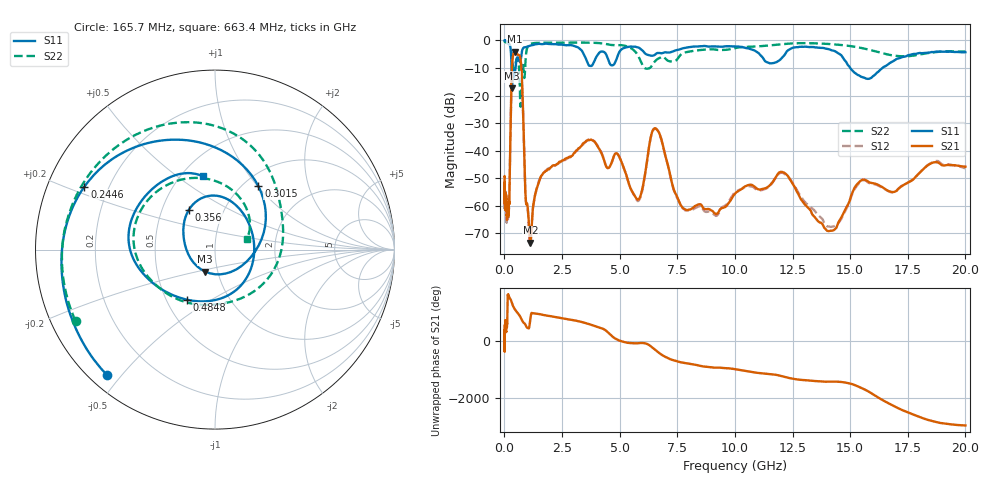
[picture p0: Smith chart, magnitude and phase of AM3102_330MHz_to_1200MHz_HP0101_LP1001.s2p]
! Date/Time: Tue, Sep 11, 2018 5:14 PM
! Network Analyzer: Agilent Technologies E8362B Rev: A.07.50.63
! Sweep from 0.010 to 20.000 GHz, 1601 Points, Sweep Type: LOG
! Power Supply: 4.949 V, 0.001 A
# Hz S DB R 50
!freq MagS11 AngS11 MagS21 AngS21 MagS12 AngS12 MagS22 AngS22
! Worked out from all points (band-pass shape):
!   1601 points, 10 MHz to 20 GHz, reference 50 ohm
!   highest |S21| = -4.09 dB at 455.8 MHz (marker M1); lowest = -73.4 dB at 1.129 GHz (marker M2)
!   |S21| within 3 dB of the highest: 347.4 MHz to 706.1 MHz (358.8 MHz wide, 68.1 % of centre)
!   lowest |S11| = -17.4 dB at 331.5 MHz (marker M3), VSWR 1.31, Z = 43.6 - j10.9 ohm
!   |S11| at or under -10 dB: 309.7 MHz to 483.4 MHz (173.8 MHz wide, 43.8 % of centre); 15.01 GHz to 16.41 GHz (1.4 GHz wide, 8.91 % of centre)
!   |S22| runs from -24.1 to -0.3 dB; largest |S21 - S12| = 0.012
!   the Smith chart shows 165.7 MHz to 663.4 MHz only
!   S11 on the Smith chart (normalised r, x): 165.7 MHz: 0.05, -0.46; 244.6 MHz: 0.11, +0.23; 301.5 MHz: 1.17, +1.01; 356 MHz: 0.68, +0.32; 484.8 MHz: 0.63, -0.39; 663.4 MHz: 0.63, +0.62
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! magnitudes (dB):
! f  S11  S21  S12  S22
! 10 MHz  0.0  -49.2  -53.5  -0.3
! 35.55 MHz  0.0  -60.4  -59.1  -0.5
! 126.4 MHz  -0.4  -64.1  -63.2  -1.0
! 165.7 MHz  -0.7  -62.3  -64.4  -1.2
! 244.6 MHz  -1.9  -43.2  -43.3  -1.8
! 301.5 MHz  -7.4  -17.4  -17.4  -3.6
! 331.5 MHz  -17.4  -9.0  -9.0  -6.4
! 356 MHz  -11.5  -6.5  -6.6  -8.3
! 447.2 MHz  -12.1  -4.1  -4.1  -9.5
! 455.8 MHz  -11.6  -4.1  -4.1  -9.2
! 484.8 MHz  -9.9  -4.2  -4.2  -8.3
! 663.4 MHz  -7.6  -5.6  -5.6  -14.5
! 925.1 MHz  -2.5  -57.4  -57.5  -6.3
! 1.129 GHz  -1.9  -73.4  -74.4  -1.3
! 1.59 GHz  -1.3  -49.3  -49.4  -0.8
! 3.757 GHz  -9.3  -36.0  -35.9  -0.8
! 5.652 GHz  -2.3  -56.4  -56.7  -3.9
! 6.549 GHz  -5.1  -31.9  -32.1  -7.4
! 7.845 GHz  -2.7  -61.4  -61.7  -4.4
! 12.09 GHz  -5.9  -47.9  -48.1  -1.3
! 14.01 GHz  -3.1  -69.1  -67.5  -1.3
! 20 GHz  -4.3  -45.8  -46.5  -4.1
